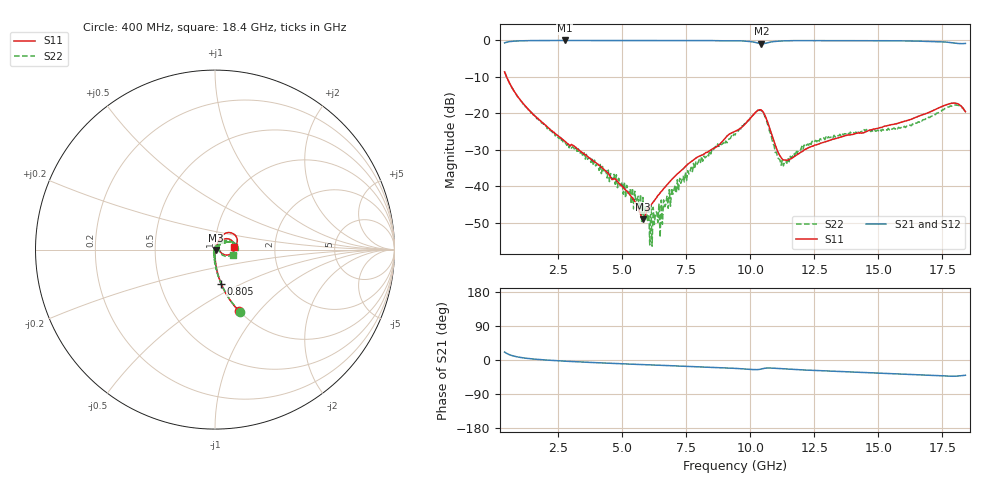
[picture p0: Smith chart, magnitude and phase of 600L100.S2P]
!  American Technical Ceramics  Date:  10/27/06
!  One Norden Lane
!  Huntington Station,  NY.  11746-2102
!  Tel:  (631) 622-4700  Fax:  (631) 622-4748
!  Part Number  600L100`	Mounting Orientation: Vertical
!  Description: Ultra Low ESR Microwave capacitors
!  Application: Coupling, Bypass, Tuning, DC Block
!  Filters, Matching
# GHZ S DB R 50
! Freq  |S11|  S11 Ph  |S21|  S21 Ph  |S12|  S12 Ph  |S22|  S22 Ph
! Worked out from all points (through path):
!   401 points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, 400 MHz to 18.4 GHz, reference 50 ohm
!   highest |S21| = -0.01 dB at 2.74 GHz (marker M1); lowest = -0.9 dB at 10.44 GHz (marker M2)
!   group delay of S21, straight-line fit = 7.48 ps
!   lowest |S11| = -49.0 dB at 5.8 GHz (marker M3), VSWR 1.01, Z = 50.3 - j0.158 ohm
!   |S11| at or under -10 dB: 480.1 MHz to end of sweep
!   |S22| runs from -56.4 to -8.6 dB; largest |S21 - S12| = 0.0018
!   S11 on the Smith chart (normalised r, x): 400 MHz: 1.00, -0.80; 805 MHz: 0.99, -0.39; 18.4 GHz: 1.23, +0.04
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0.4  -8.62 -68.4  -0.68 21.0  -0.68 21.1  -8.60 -68.4
0.805  -14.30 -79.8  -0.18 9.5  -0.18 9.5  -14.40 -80.1
1.525  -20.30 -86.5  -0.05 2.6  -0.05 2.5  -20.48 -86.6
2.74  -27.59 -91.0  -0.01 -3.0  -0.02 -3.0  -27.82 -95.4
3.415  -30.61 -91.2  -0.02 -5.4  -0.02 -5.4  -30.87 -93.4
5.125  -40.96 -74.0  -0.02 -10.3  -0.02 -10.3  -43.17 -114.8
5.8  -49.04 -26.3  -0.04 -12.2  -0.04 -12.2  -43.04 -164.1
6.025  -45.69 9.3  -0.03 -12.7  -0.03 -12.7  -45.42 -163.1
6.07  -45.44 11.5  -0.03 -12.8  -0.03 -12.8  -56.04 150.1
6.43  -42.21 32.7  -0.03 -13.8  -0.03 -13.8  -44.86 135.3
6.475  -41.78 34.6  -0.03 -13.9  -0.03 -13.9  -53.96 101.5
7.015  -37.50 49.1  -0.03 -15.4  -0.03 -15.4  -41.12 73.8
7.78  -32.75 56.8  -0.04 -17.4  -0.04 -17.4  -33.71 70.5
9.4  -24.91 56.5  -0.11 -22.1  -0.11 -22.1  -25.92 50.8
10.435  -19.13 4.0  -0.91 -23.6  -0.91 -23.6  -19.33 -3.0
11.2  -32.10 -7.3  -0.16 -22.9  -0.15 -22.9  -34.20 -3.2
11.515  -32.68 22.6  -0.09 -24.2  -0.09 -24.2  -33.26 35.1
12.415  -29.01 51.7  -0.05 -27.3  -0.04 -27.3  -27.63 53.1
15.43  -23.20 65.5  -0.10 -35.7  -0.09 -35.8  -24.51 40.6
16.285  -21.62 64.2  -0.16 -38.3  -0.16 -38.3  -23.39 34.5
17.815  -17.29 38.4  -0.57 -42.8  -0.57 -42.8  -17.93 11.5
18.4  -19.53 9.3  -0.82 -40.3  -0.82 -40.4  -19.56 -17.7
